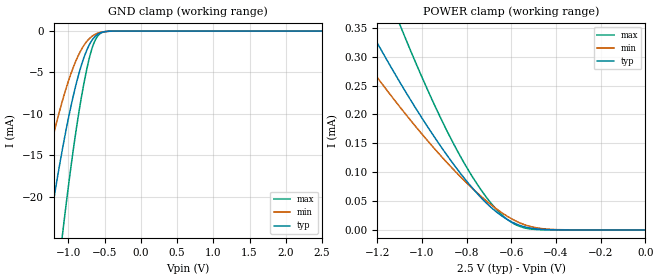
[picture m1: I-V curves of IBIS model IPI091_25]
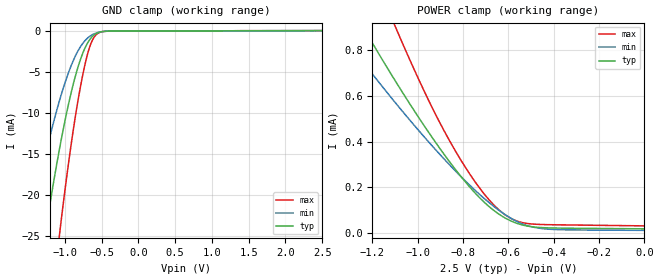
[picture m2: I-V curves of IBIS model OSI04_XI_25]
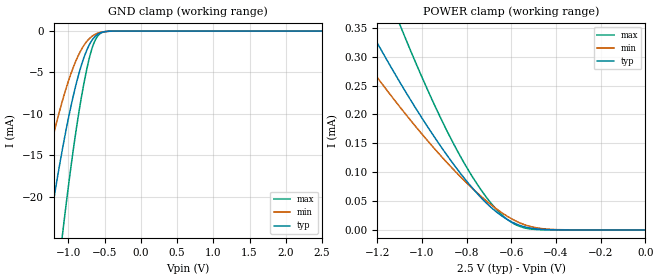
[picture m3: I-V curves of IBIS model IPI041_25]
| TEXAS INSTRUMENTS INCORPORATED
| Connectivity Solutions Group
| IBIS Model of TL16C550DZQS_2.5V
| 550D_ZQS_2.5V
| This file contains package information for the following:
|  ZQS 24-pin (BGA) package as [Component] 550DZQS_2.5V
| This device can be powered at the following Vccs:
|  2.5 Volt Vcc
| This file provides unique models under the [Model Selector] for each Vcc.
| For operation at a specific Vcc, select the appropriate model after each
| [Model Selector] keyword.
[IBIS Ver]   3.2
[Comment char]  |_char
[File Name]   550D_ZQS_2.5V.ibs
[File Rev]   1 | a
[Date]   December 15, 2008
[Source]   Data created from TI-SPICE simulations at TI-CONN.
[Notes]   The following is an IBIS list for the 550D_ZQS_2.5V.
   Please contact s-ly@ti.com with questions and
   comments concerning CONN IBIS models.
[Disclaimer] Property of Texas Instruments Incorporated.  Unauthorized
   reproduction and/or distribution is strictly prohibited.
   This product is protected under copyright law.
   Created  2003, (C) Copyright  2003, Texas Instruments
   Incorporated, All Rights Reserved
   UNLESS THERE IS A SIGNED, WRITTEN AGREEMENT TO THE
   CONTRARY, TEXAS INSTRUMENTS (TI) IS PROVIDING THE IBIS
   MODELS  AND WITHOUT ANY WARRANTY, EXPRESSED OR
   IMPLIED.  TI assumes no liability for:
   1) the accuracy of the IBIS models provided to your
   company;
   2) the proper functioning of these IBIS Models in your
   design or for any resulting applications; or
   3) infringement of patents, copyrights or intellectual
   property rights resulting from your use of these IBIS
   models.
   TI provides IBIS Models as a service to our customers.
   You and your company shall not distribute, sell or give
   these models to anyone else without prior written
   permission from TI.
   TI reserves the right to make changes to our products or
   to discontinue any semiconductor product or service
   without notice, and advises our customers to obtain the
   latest version of relevant information to verify, before
   placing orders, that the information being relied on is
   current.
   Please be aware that your receipt and use of the IBIS
   information provided shall serve as acceptance of these
   terms and conditions.  If you do not accept these terms,
   you should return or destroy the IBIS models and any
   other accompanying information immediately.
| Component 550D_2.5V_ZQS 24-pin BGA
[Component]   550D_ZQS_2.5V
[Manufacturer]   Texas Instruments, Inc.
[Package]
|   typ   min   max
R_pkg   4.665e-02   3.264e-02   6.067e-02
L_pkg   1.009e-09   0.683e-09   1.336e-09
C_pkg   2.424e-13   1.463e-13   3.850e-13
[Pin]   signal_name   model_name   R_pin   L_pin   C_pin
A1   D5   IPI04_OPJ43   3.914e-02   0.909e-09   1.463e-13
A2   D4   IPI04_OPJ43   3.358e-02   0.717e-09   1.685e-13
A3   D2   IPI04_OPJ43   3.418e-02   0.721e-09   1.686e-13
A4   D0   IPI04_OPJ43   3.779e-02   0.849e-09   1.744e-13
A5   VCC   POWER   4.675e-02   1.160e-09   1.698e-13
B1   D7   IPI04_OPJ43   3.408e-02   0.733e-09   1.672e-13
B3   D3   IPI04_OPJ43   4.552e-02   0.909e-09   3.306e-13
B4   D1   IPI04_OPJ43   4.866e-02   1.034e-09   3.084e-13
B5   MR   IPI091   3.264e-02   0.686e-09   1.664e-13
C1   SIN   IPI041   3.268e-02   0.683e-09   1.584e-13
C2   SOUT   OPJ430   4.586e-02   0.916e-09   3.238e-13
C3   D6   IPI04_OPJ43   5.719e-02   1.336e-09   3.850e-13
C4   CTSB   IPI041   6.067e-02   1.225e-09   3.274e-13
C5   RTSB   OPJ430   3.287e-02   0.693e-09   1.555e-13
D1   CS2B   IPI041   3.303e-02   0.701e-09   1.630e-13
D2   WR1B   IPI041   4.588e-02   0.923e-09   2.961e-13
D3   RD1B   IPI041   4.627e-02   0.925e-09   3.222e-13
D4   INTRPT   OPJ430   4.611e-02   0.954e-09   2.955e-13
D5   A0   IPI041   3.389e-02   0.724e-09   1.619e-13
E1   XIN   OSI04_XI   3.991e-02   0.937e-09   1.534e-13
E2   XOUT   OSI04   3.400e-02   0.722e-09   1.635e-13
E3   VSS   GND   3.336e-02   0.700e-09   1.624e-13
E4   A2   IPI041   3.740e-02   0.828e-09   1.710e-13
E5   A1   IPI041   4.103e-02   0.969e-09   1.494e-13
| Model IPI091
[Model Selector]   IPI091
IPI091_25   2.5 volt Vcc
| Model OSI04_XI
[Model Selector]   OSI04_XI
OSI04_XI_25   2.5 volt Vcc
| Model IPI041
[Model Selector]   IPI041
IPI041_25   2.5 volt Vcc
| Model IPI04_OPJ43
[Model Selector]   IPI04_OPJ43
IPI04_OPJ43_25   2.5 volt Vcc
| Model OPJ430
[Model Selector]   OPJ430
OPJ430_25   2.5 volt Vcc
| Model OSI04
[Model Selector]   OSI04
OSI04_25   2.5 volt Vcc
| Models and submodels in the file (6): IPI091_25 (Input), OSI04_XI_25 (Input), IPI041_25 (Input), IPI04_OPJ43_25 (I/O), OPJ430_25 (3-state), OSI04_25 (3-state)
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[Model]   IPI091_25
Model_type  Input
Vinl = 0
Vinh = 2.5
| variable   typ   min   max
C_comp   1.09pF   0.97pF   1.21pF
[Temperature Range]   40   125   -40
| Ambient temperature   25   110   -40
[Voltage range]   2.5   2.3   2.7
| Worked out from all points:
|   GND clamp passes 1 mA (typ) near -0.66 V on its own axis
|   POWER clamp passes 1 mA (typ) near -2.03 V on its own axis
[GND Clamp]
| IPI091_25
|   Voltage   I(typ)   I(min)   I(max)
-2.5V     -115mA     -79.72mA   -164.4mA
-1.485V   -37.43mA   -23.94mA   -59.12mA
-1.265V   -23.92mA   -14.77mA   -39.38mA
-1.08V    -14.2mA    -8.377mA   -24.56mA
-1.065V   -13.5mA    -7.923mA   -23.45mA
-955mV    -8.737mA   -4.937mA   -15.83mA
-830mV    -4.417mA   -2.392mA   -8.532mA
-730mV    -2.005mA   -1.091mA   -3.99mA
-635mV    -690.9uA   -415.3uA   -1.203mA
-560mV    -221.4uA   -161.8uA   -300.1uA
-440mV    -21.14uA   -26.42uA   -19.38uA
2.5V      179.9pA    7.156nA    49.54pA
[POWER Clamp]
| IPI091_25
|   Voltage   I(typ)   I(min)   I(max)
-2.5V     1.454mA    1.097mA    2.083mA
-1.36V    439.4uA    350.2uA    624.8uA
-1.235V   348.4uA    282.4uA    491.3uA
-1.095V   253.5uA    211.2uA    352uA
-1.075V   240.6uA    201.5uA    333.1uA
-945mV    161.4uA    141.3uA    217.5uA
-830mV    99.28uA    93.13uA    129uA
-720mV    49.87uA    53.05uA    61.07uA
-630mV    21.07uA    26.64uA    21.99uA
-550mV    6.466uA    10.43uA    4.583uA
-465mV    1.046uA    2.442uA    370.2nA
-31.11fV  179.9pA    1.684nA    54.24pA
[Model]   OSI04_XI_25
Model_type  Input
Vinl = 0
Vinh = 2.5
| variable   typ   min   max
C_comp   1.81pF   1.12pF   2.40pF
[Temperature Range]   40   125   -40
| Ambient temperature   25   110   -40
[Voltage range]   2.5   2.3   2.7
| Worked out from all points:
|   GND clamp passes 1 mA (typ) near -0.66 V on its own axis
|   POWER clamp passes 1 mA (typ) near -1.30 V on its own axis
[GND Clamp]
| OSI04_XI_25
|   Voltage   I(typ)   I(min)   I(max)
-2.5V     -117.2mA   -81mA      -167.9mA
-1.48V    -38.04mA   -24.27mA   -60.11mA
-1.26V    -24.32mA   -15mA      -40.01mA
-1.075V   -14.44mA   -8.535mA   -24.92mA
-1.06V    -13.72mA   -8.076mA   -23.8mA
-930mV    -8.097mA   -4.582mA   -14.76mA
-815mV    -4.206mA   -2.33mA    -8.111mA
-710mV    -1.776mA   -1.037mA   -3.434mA
-625mV    -669.3uA   -465.2uA   -1.116mA
-545mV    -205.3uA   -194.2uA   -270.4uA
-430mV    -40.49uA   -47uA      -53.13uA
2.5V      19.05uA    13.35uA    29.56uA
[POWER Clamp]
| OSI04_XI_25
|   Voltage   I(typ)   I(min)   I(max)
-2.5V     3.431mA    2.617mA    4.916mA
-1.355V   1.099mA    896.3uA    1.535mA
-1.24V    898.6uA    746.4uA    1.242mA
-1.22V    864.6uA    720.9uA    1.193mA
-1.095V   659.2uA    565.9uA    893.7uA
-935mV    416.4uA    380.2uA    546.2uA
-830mV    273.7uA    268.3uA    352.9uA
-720mV    148uA      163.2uA    188uA
-625mV    72.54uA    88.13uA    88.07uA
-555mV    40.52uA    47.83uA    50.59uA
-465mV    25.13uA    21.75uA    38.3uA
-31.11fV  19.05uA    12.27uA    31.94uA
[Model]   IPI041_25
Model_type  Input
Vinl = 0
Vinh = 2.5
| variable   typ   min   max
C_comp   1.10pF   0.98pF   1.21pF
[Temperature Range]   40   125   -40
| Ambient temperature   25   110   -40
[Voltage range]   2.5   2.3   2.7
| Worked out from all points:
|   GND clamp passes 1 mA (typ) near -0.66 V on its own axis
|   POWER clamp passes 1 mA (typ) near -2.03 V on its own axis
[GND Clamp]
| IPI041_25
|   Voltage   I(typ)   I(min)   I(max)
-2.5V     -115mA     -79.72mA   -164.4mA
-1.485V   -37.43mA   -23.94mA   -59.12mA
-1.265V   -23.92mA   -14.77mA   -39.38mA
-1.08V    -14.2mA    -8.377mA   -24.56mA
-1.065V   -13.5mA    -7.923mA   -23.45mA
-955mV    -8.737mA   -4.937mA   -15.83mA
-830mV    -4.417mA   -2.392mA   -8.532mA
-730mV    -2.005mA   -1.091mA   -3.99mA
-635mV    -690.9uA   -415.3uA   -1.203mA
-560mV    -221.4uA   -161.8uA   -300.1uA
-440mV    -21.14uA   -26.42uA   -19.38uA
2.5V      179.9pA    7.156nA    49.54pA
[POWER Clamp]
| IPI041_25
|   Voltage   I(typ)   I(min)   I(max)
-2.5V     1.454mA    1.097mA    2.083mA
-1.36V    439.4uA    350.2uA    624.8uA
-1.235V   348.4uA    282.4uA    491.3uA
-1.095V   253.5uA    211.2uA    352uA
-1.075V   240.6uA    201.5uA    333.1uA
-945mV    161.4uA    141.3uA    217.5uA
-830mV    99.28uA    93.13uA    129uA
-720mV    49.87uA    53.05uA    61.07uA
-630mV    21.07uA    26.64uA    21.99uA
-550mV    6.466uA    10.43uA    4.583uA
-465mV    1.046uA    2.442uA    370.2nA
-31.11fV  179.9pA    1.684nA    54.24pA
